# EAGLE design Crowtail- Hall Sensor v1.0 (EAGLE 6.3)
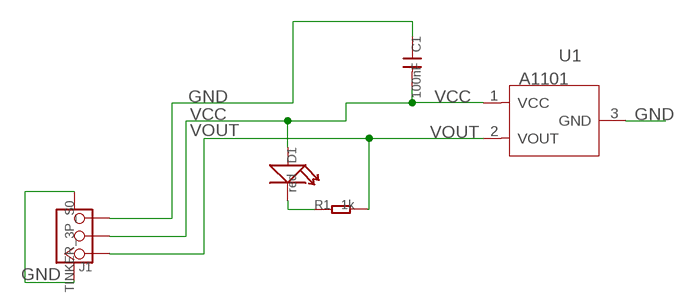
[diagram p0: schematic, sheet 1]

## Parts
C1  100nF  C-0603  [0603]
D1  red  LED'0603'  [LED-0603]
J1  TINKER_3P_S0  [TINKER_3P_S0]
R1  1k  R-0603  [R0603]
U1  A1101  [SOT-23W]

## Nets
GND: C1.1 J1.3 J1.SS1 J1.SS2 U1.3(GND)
N$1: D1.- R1.1
VCC: C1.2 D1.+ J1.2 U1.1(VCC)
VOUT: J1.1 R1.2 U1.2(VOUT)

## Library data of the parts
C1 = Discrete:C*: Ceramic Capacitors
D1 = Discrete:LED*
J1 = Connector:TINKER_3P_S0
R1 = Discrete:R*
U1 = IC:A1101: Continuous-Time Switch

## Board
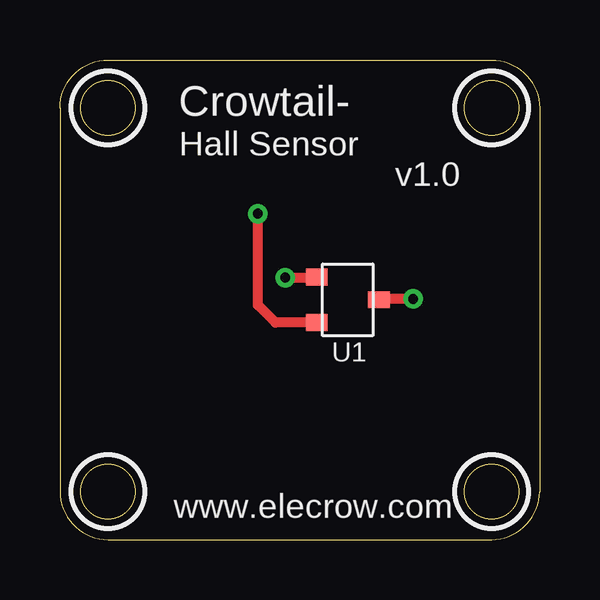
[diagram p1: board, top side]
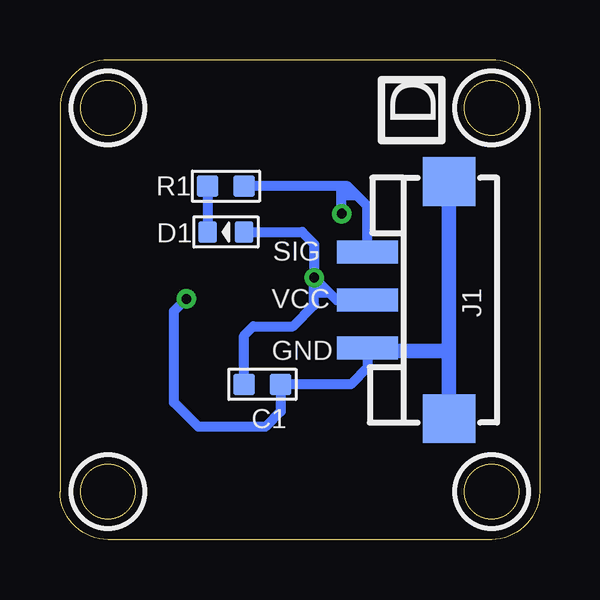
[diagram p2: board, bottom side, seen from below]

Size 20 x 20 mm. Coordinates in mm from the lower left corner, seen from the top.
Outline: 0,18 0,2 arc90 2,0 18,0 arc90 20,2 20,18 arc90 18,20 2,20 arc90 0,18
Outline: circle at 2,18 radius 1.14
Outline: circle at 2,2 radius 1.14
Outline: circle at 18,18 radius 1.14
Outline: circle at 18,2 radius 1.14
Copper layers (1*16): Top 0.035mm / dielectric 1.5mm / Bottom 0.035mm
Design rules "default *": minimum track width 10mil, minimum drill 24mil, track to track 8mil, track to pad 8mil, pad to pad 8mil, via to via 8mil, smd to smd 8mil, copper to edge 40mil, drill to drill 8mil, minimum pad ring 10mil, minimum via ring 8mil, stop-mask expansion 2mil, vias tented up to drill 100mil, thermal gap 10mil
tRestrict: area 0.5,16.5 to 3.5,19.5; area 0.5,0.5 to 3.5,3.5; area 16.5,16.5 to 19.5,19.5; area 16.5,0.5 to 19.5,3.5
bRestrict: area 0.5,16.5 to 3.5,19.5; area 0.5,0.5 to 3.5,3.5; area 16.5,16.5 to 19.5,19.5; area 16.5,0.5 to 19.5,3.5

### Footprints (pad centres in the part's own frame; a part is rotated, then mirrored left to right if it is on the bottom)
0603 = smd 0.889 x 0.889: 1 -0.762,0; 2 0.762,0
LED-0603 = smd 0.762 x 0.889: + -0.762,0; - 0.762,0
TINKER_3P_S0 = smd 0.965 x 2.54: 1 -1.984,-3.175; 2 0.016,-3.175; 3 2.016,-3.175 | smd 2.032 x 2.184: SS1 -4.93,0.225; SS2 4.962,0.225
R0603 = smd 0.889 x 0.889: 1 -0.762,0; 2 0.762,0
SOT-23W = smd 0.7 x 0.9: 1 -0.95,-1.3; 2 0.95,-1.3; 3 0,1.3

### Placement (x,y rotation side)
C1  11.56,6.48 180 bottom
D1  13.08,12.83 180 bottom
J1  4,10 270 bottom
R1  13.08,14.73 0 bottom
U1  12,10 270 top

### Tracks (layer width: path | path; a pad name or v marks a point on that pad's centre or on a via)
GND  (via drill 0.41 pad 0.3)
  Top 0.406: v14.73,10.03 13.33,10.03 U1.3
  Bottom 0.406: J1.3 7.17,7.18 7.87,6.48 C1.1 10.79,5.33 11.43,4.7 14.22,4.7 15.24,5.71 15.24,9.53 v14.73,10.03
  Bottom 0.61: J1.SS1 J1.SS2 3.77,7.84 3.81,7.87 7.07,7.87 J1.3
N$1
  Bottom 0.406: R1.1 D1.-
N$3
  Bottom 0.406: 7.75,14.35 8.13,14.35
N$4
  Bottom 0.406: 8.89,10.29 9.27,10.29
VCC  (via drill 0.41 pad 0.3)
  Top 0.406: v9.4,10.92 10.67,10.92 U1.1
  Bottom 0.406: J1.2 8.46,9.98 v9.4,10.92 | C1.2 12.32,8.51 11.94,8.89 10.29,8.89 9.4,9.78 v9.4,10.92 | D1.+ 9.91,12.83 9.4,12.32 v9.4,10.92
VOUT  (via drill 0.41 pad 0.3)
  Top 0.406: U1.2 8.98,9.05 8.26,9.78 v8.26,13.59
  Bottom 0.406: J1.1 7.17,13.91 8,14.73 8.26,14.73 | 8.26,14.73 R1.2 | v8.26,13.59 8.26,14.73

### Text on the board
tPlace: Crowtail- | Hall Sensor | v1.0 | www.elecrow.com
bPlace: D | SIG | VCC | GND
